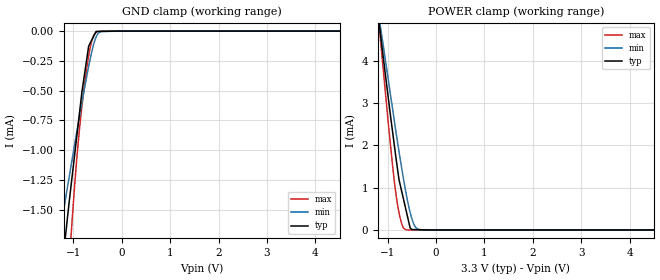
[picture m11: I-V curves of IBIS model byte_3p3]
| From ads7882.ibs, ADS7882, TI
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|   byte_3p3 Model
[Model]   byte_3p3
Model_type   Input
Vinl = 0.8
Vinh = 2.3
|   typ   min   max
|   (nom PVT)   (Fast PVT)   (slow PVT)
|C_comp from frequency sweep method (F=1.5MHz)
|Average
C_comp   2.550e-12   2.457e-12   2.647e-12
|C_comp from LC tank measurement(L=1nH)
|Resonant Frequency(Hz)   3.600e+09   3.650e+09   3.520e+09
|C_comp   1.956e-12   1.903e-12   2.046e-12
| Where nom  PVT is Nominal Process,  3.3V,  25C
|   Fast PVT is Strong Process,   3.6V,  -40C
|   Slow PVT is Weak Process,   3V,  85C
[Model Spec]
Vinh   2.3   2   2.6
[Voltage Range]   3.3   3   3.6
|Ambient Temperature   25   85   -40
|Junction Temperature
[Temperature Range]   25   85   -40
[Power Clamp Reference]   3.3   3   3.6
[GND Clamp Reference]   0   0   0
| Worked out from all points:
|   GND clamp passes 1 mA (typ) near -0.97 V on its own axis
|   POWER clamp passes 1 mA (typ) near -0.73 V on its own axis
[GND Clamp]
|   Voltage   I(typ)   I(min)   I(max)
-3.3V     -9.969mA   -6.836mA   -17.31mA
-1.392V   -2.567mA   -1.972mA   -3.928mA
-1.183V   -1.786mA   -1.455mA   -2.546mA
-1.14V    -1.624mA   -1.348mA   -2.278mA
-1.089V   -1.433mA   -1.224mA   -1.962mA
-1.032V   -1.233mA   -1.085mA   -1.608mA
-873.6mV  -678.1uA   -709.9uA   -809.9uA
-729.6mV  -245.6uA   -385.9uA   -321uA
-643.2mV  -91.81uA   -212.7uA   -117.8uA
-534.6mV  -3.685uA   -51.42uA   -12.39uA
0V        0A         0A         0A
6.6V      0A         0A         0A
[POWER Clamp]
|   Voltage   I(typ)   I(min)   I(max)
-3.3V     25.73mA    22.48mA    32.55mA
-1.356V   6.604mA    6.48mA     7.124mA
-1.147V   4.613mA    4.794mA    4.476mA
-992.4mV  3.167mA    3.59mA     2.581mA
-823.2mV  1.657mA    2.276mA    798.9uA
-765.6mV  1.188mA    1.853mA    408.5uA
-711.6mV  919.6uA    1.47mA     151.9uA
-614.4mV  437.1uA    832.1uA    2.79uA
-534.6mV  41.03uA    406.5uA    657.4nA
-459mV    8.184uA    134.1uA    0A
-270mV    3.926uA    19.11nA    0A
6.6V      0A         0A         0A
